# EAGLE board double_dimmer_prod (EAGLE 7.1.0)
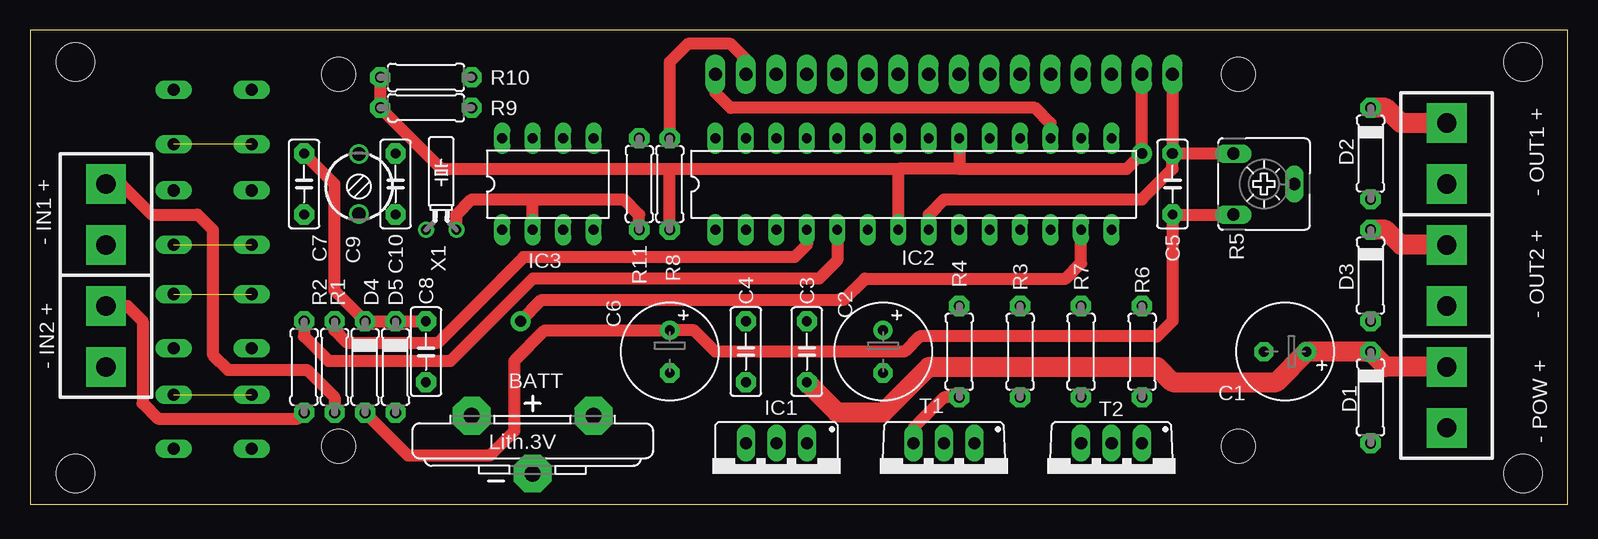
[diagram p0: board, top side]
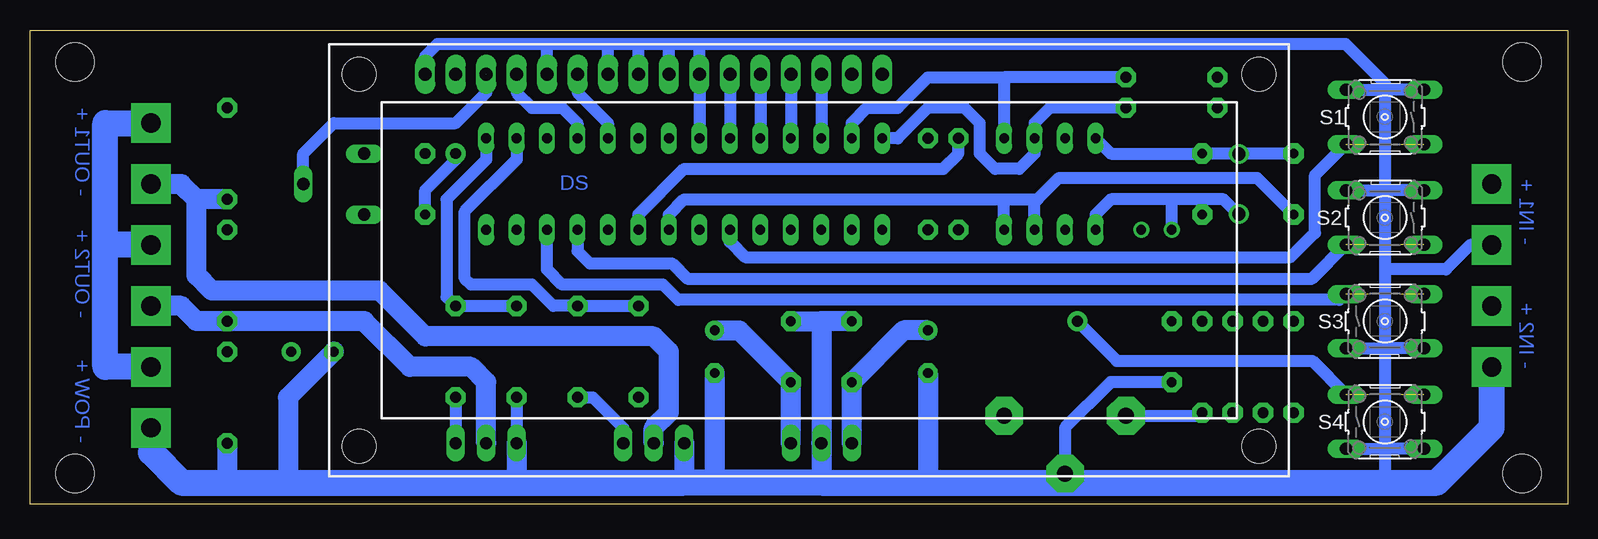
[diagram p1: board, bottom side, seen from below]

Size 128.18 x 39.51 mm. Coordinates in mm from the lower left corner, seen from the top.
Outline: 128.18,0 128.18,39.51 0,39.51 0,0 128.18,0
Copper layers (1*16): Top 0.035mm / dielectric 1.5mm / Bottom 0.035mm
Design rules "default": minimum track width 10mil, minimum drill 24mil, track to track 8mil, track to pad 8mil, pad to pad 8mil, via to via 8mil, smd to smd 8mil, copper to edge 40mil, drill to drill 8mil, minimum pad ring 10mil, minimum via ring 8mil, stop-mask expansion 4mil, vias tented up to drill 0mil, thermal gap 10mil
Holes 3.2 mm at 3.8,36.83 3.8,2.54 124.45,2.54 124.45,36.83

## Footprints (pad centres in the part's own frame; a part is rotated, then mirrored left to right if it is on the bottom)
CR2032V = drill 1.321 pad 3.15 octagon: + -2.54,-5.08; +@1 -2.54,5.08; - 2.286,0
E3,5-8 = drill 0.813 pad 1.6: + -1.778,0 | drill 0.813 pad 1.6 octagon: - 1.778,0
C050-025X075 = drill 0.813 pad 1.676 octagon: 1 -2.54,0; 2 2.54,0
CTRIM3050.504 = drill 1.1: 1 -2.5,0; 2 2.5,0
0207/7 = drill 0.9 pad 1.676 octagon: 1 -3.81,0; 2 3.81,0
78XXS = drill 1.016 long: GND 0,-2.54; IN -2.54,-2.54; OUT 2.54,-2.54
DIL28-3 = drill 0.813 long: 1 -16.51,-3.81; 2 -13.97,-3.81; 3 -11.43,-3.81; 4 -8.89,-3.81; 5 -6.35,-3.81; 6 -3.81,-3.81; 7 -1.27,-3.81; 8 1.27,-3.81; 9 3.81,-3.81; 10 6.35,-3.81; 11 8.89,-3.81; 12 11.43,-3.81; 13 13.97,-3.81; 14 16.51,-3.81; 15 16.51,3.81; 16 13.97,3.81; 17 11.43,3.81; 18 8.89,3.81; 19 6.35,3.81; 20 3.81,3.81; 21 1.27,3.81; 22 -1.27,3.81; 23 -3.81,3.81; 24 -6.35,3.81; 25 -8.89,3.81; 26 -11.43,3.81; 27 -13.97,3.81; 28 -16.51,3.81
DIL08 = drill 0.813 long: 1 -3.81,-3.81; 2 -1.27,-3.81; 3 1.27,-3.81; 4 3.81,-3.81; 5 3.81,3.81; 6 1.27,3.81; 7 -1.27,3.81; 8 -3.81,3.81
LCD-16X2 = drill 1.1 long: 1 -32,15.5; 2 -29.46,15.5; 3 -26.92,15.5; 4 -24.38,15.5; 5 -21.84,15.5; 6 -19.3,15.5; 7 -16.76,15.5; 8 -14.22,15.5; 9 -11.68,15.5; 10 -9.14,15.5; 11 -6.6,15.5; 12 -4.06,15.5; 13 -1.52,15.5; 14 1.02,15.5; 15 3.56,15.5; 16 6.1,15.5 | hole 2.8: -37.5,15.5; -37.5,-15.5; 37.5,15.5; 37.5,-15.5
CA6V = drill 1.016 long: A -2.54,-2.54; E 2.54,-2.54; S 0,2.54
B3F-10XX = drill 1.016 long: 1 -3.251,2.261; 2 3.251,2.261; 3 -3.251,-2.261; 4 3.251,-2.261
TO220BV = drill 1.016 long: D 0,-2.54; G -2.54,-2.54; S 2.54,-2.54
TC26H = drill 0.813: 1 -1.27,0; 2 1.27,0

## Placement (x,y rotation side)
BATT  [CR2032V]  41.9,4.83 270 top
C1  220uF  [E3,5-8]  104.64,12.7 180 top
C2  220uF  [E3,5-8]  71.11,12.7 270 top
C3  100nF  [C050-025X075]  64.76,12.7 90 top
C4  100nF  [C050-025X075]  59.68,12.7 90 top
C5  100nF  [C050-025X075]  95.24,26.67 90 top
C6  220uF  [E3,5-8]  53.33,12.7 270 top
C7  100nF  [C050-025X075]  22.85,26.67 270 top
C8  100nF  [C050-025X075]  33.01,12.7 270 top
C9  22pF  [CTRIM3050.504]  27.42,26.67 270 top
C10  22pF  [C050-025X075]  30.47,26.67 270 top
D1  1N5819  [0207/7]  111.75,8.89 90 top
D2  1N5819  [0207/7]  111.75,29.21 90 top
D3  1N5819  [0207/7]  111.75,19.05 90 top
D4  1N5819  [0207/7]  27.93,11.43 270 top
D5  1N5819  [0207/7]  30.47,11.43 270 top
IC1  7805  [78XXS]  62.22,2.54 180 top
IC2  ATMEGA8  [DIL28-3]  73.65,26.67 0 top
IC3  PFC8583  [DIL08]  43.17,26.67 0 top
IC4  LCD2x16  [LCD-16X2]  63.24,20.32 0 bottom
R1  3.3k  [0207/7]  25.39,11.43 270 top
R2  3.3k  [0207/7]  22.85,11.43 270 top
R3  47R  [0207/7]  82.54,12.7 90 top
R4  3.3k  [0207/7]  77.46,12.7 90 top
R5  10k  [CA6V]  102.86,26.67 270 top
R6  47R  [0207/7]  92.7,12.7 90 top
R7  3.3k  [0207/7]  87.62,12.7 90 top
R8  47R  [0207/7]  53.33,26.67 270 top
R9  3.3k  [0207/7]  33.01,33.02 0 top
R10  3.3k  [0207/7]  33.01,35.56 0 top
R11  1M  [0207/7]  50.79,26.67 270 top
S1  [B3F-10XX]  15.23,32.26 180 bottom
S2  [B3F-10XX]  15.23,23.88 180 bottom
S3  [B3F-10XX]  15.23,15.24 0 bottom
S4  [B3F-10XX]  15.23,6.86 0 bottom
T1  [TO220BV]  76.19,2.54 180 top
T2  [TO220BV]  90.16,2.54 180 top
X1  32kHz  [TC26H]  34.28,22.86 0 top

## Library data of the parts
BATT = battery
C1-C10 D1-D5 R1-R4 R6-R11 = rcl
IC1 = v-reg
IC2 = avr-4
IC3 = micro-philips; OC_FARNELL: unknown; OC_NEWARK: unknown
IC4 = moja2
R5 = pot
S1-S4 = switch-omron; MPN: B3F-1000; OC_FARNELL: 176432; OC_NEWARK: 36M3542
T1 T2 = transistor-power
X1 = crystal; OC_FARNELL: unknown; OC_NEWARK: unknown

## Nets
32K: IC2.9 R11.1
BKL: IC2.17 IC4.16
D4: IC2.23 IC4.11
D5: IC2.24 IC4.12
D6: IC2.25 IC4.13
D7: IC2.26 IC4.14
EIN1: IC2.4 R1.1
EIN2: IC2.5 R2.1
EN: IC2.19 IC4.6
GND: BATT.- C1.- C2.- C3.2 C4.2 C5.2 C6.- C7.2 C8.2 D1.1 IC1.GND IC2.8 IC2.22 IC3.3 IC3.4 IC4.1 IC4.5 IC4.7 IC4.8 IC4.9 IC4.10 R4.1 R5.A R7.1 S1.3 S1.4 S2.3 S2.4 S3.3 S3.4 S4.3 S4.4 T1.S T2.S
N$1: R6.1 T2.G
N$2: D2.1 T1.D
N$3: IC4.3 R5.S
N$4: D3.1 T2.D
N$5: R3.1 T1.G
N$6: BATT.+ D5.2
N$7: IC4.15 R8.1
N$8: C9.2 C10.2 IC3.1 X1.1
N$9: R2.2
N$10: IC3.2 R11.2 X1.2
N$11: R1.2
N$40: C7.1 C8.1 C9.1 C10.1 D4.1 D5.1 IC3.8
OT1: IC2.16 R3.2 R4.2
OT2: IC2.15 R6.2 R7.2
RS: IC2.18 IC4.4
RXD: IC2.2
SCL: IC2.28 IC3.6 R9.2
SDA: IC2.27 IC3.5 R10.2
SW1: IC2.6 S1.1 S1.2
SW2: IC2.11 S2.1 S2.2
SW3: IC2.12 S3.1 S3.2
SW4: IC2.13 S4.1 S4.2
TXD: IC2.3
VCC: C1.+ C2.+ C3.1 D1.2 D2.2 D3.2 IC1.IN
VDD: C4.1 C5.1 C6.+ D4.2 IC1.OUT IC2.7 IC2.20 IC4.2 R5.E R8.2 R9.1 R10.1

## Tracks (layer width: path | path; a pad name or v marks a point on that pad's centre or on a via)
32K
  Bottom 1.016: IC2.9 77.46,24.13 73.65,27.94 52.06,27.94 50.79,29.21 R11.1
BKL
  Top 1.016: IC2.17 85.08,31.75 83.81,33.02 58.41,33.02 57.14,34.29 IC4.16
D4
  Bottom 1.016: IC4.11 IC2.23
D5
  Bottom 1.016: IC4.12 IC2.24
D6
  Bottom 1.016: IC4.13 IC2.25
D7
  Bottom 1.016: IC4.14 IC2.26
EIN1
  Top 1.016: R1.1 25.39,14.48 26.41,13.46 34.03,13.46 41.14,20.57 63.74,20.57 64.76,21.59 IC2.4
EIN2
  Top 1.016: R2.1 22.85,13.97 24.88,11.94 35.04,11.94 41.9,18.8 65.78,18.8 67.3,20.32 IC2.5
EN
  Bottom 1.016: IC4.6 82.54,34.29 80,31.75 IC2.19
GND  (via drill 0.9 pad 1.68, 1.6 pad 3.3)
  Top 1.016: R5.A C5.2 | IC4.1 C5.2 95.24,27.94 92.69,25.4 76.19,25.4 74.92,24.13 IC2.8 | R4.1 76.19,8.89 73.65,6.35 T1.S
  Bottom 1.016: 15.23,34.8 15.23,35.05 18.53,38.35 72.38,38.35 | 15.23,34.8 15.23,26.16 | 15.23,26.16 15.23,25.91 | 15.23,25.91 15.23,19.56 | 15.23,19.56 15.23,13.21 | 15.23,13.21 15.23,12.95 | 15.23,12.95 15.23,4.57 | 15.23,4.57 15.23,4.32 | 15.23,4.32 15.23,2.03 14.98,1.78 | S3.3 15.46,12.98 15.23,13.21 | S3.4 15.21,12.98 15.23,12.95 | S4.4 15.21,4.6 15.23,4.57 | S4.3 15.51,4.6 15.23,4.32 | 72.38,38.35 IC4.10 IC2.22 | IC4.7 80,38.1 | 80,38.1 80,38.35 77.46,38.35 | 77.46,38.35 74.92,38.35 | 74.92,38.35 72.38,38.35 | IC4.9 74.92,38.35 | IC4.8 77.46,38.35 | IC4.1 95.24,37.33 94.22,38.35 85.08,38.35 | 85.08,38.35 80.25,38.35 80,38.1 | IC4.5 85.08,38.35 | C5.2 | R7.1 T2.S | C7.2 25.9,27.18 42.41,27.18 44.19,25.4 44.44,25.4 | S1.3 14.95,34.52 15.23,34.8 | S1.4 15.51,34.52 15.23,34.8 | S2.3 15,26.14 15.23,25.91 | S2.4 15.25,26.14 15.23,26.16 | C8.2 38.09,10.16 41.9,6.35 BATT.- | v6.34,21.59 8.12,21.59 10.15,19.56 15.23,19.56 | IC2.8 74.92,24.13 73.65,25.4 46.98,25.4 | 46.98,25.4 44.44,25.4 | IC3.3 44.44,25.4 | IC3.4 46.98,25.4
  Bottom 1.676: 62.22,1.78 IC1.GND 62.22,15.24 | T1.S 73.65,1.78 | T2.S 87.62,1.78 | D1.1 111.75,1.78 | C1.- 106.67,8.89 106.67,2.03 106.92,1.78 | C2.- 71.11,1.78 | C3.2 62.22,15.24 | C4.2 62.22,15.24 | C6.- 53.33,1.78
  Bottom 2.184: v118.1,6.35 118.1,4.32 115.56,1.78 111.75,1.78 106.92,1.78 87.62,1.78 73.65,1.78 71.11,1.78 62.22,1.78 53.33,1.78 41.9,1.78 | 41.9,1.78 14.98,1.78 10.91,1.78 6.34,6.35 v6.34,11.43 | BATT.- 41.9,1.78
  other vias: 95.24,29.21
N$1
  Bottom 1.016: R6.1 T2.G
N$2  (via drill 1.6 pad 3.3)
  Bottom 1.676: T1.D 76.19,6.35 74.92,7.62 74.92,12.7 76.19,13.97 95.24,13.97 99.05,17.78 113.02,17.78 114.29,19.05 114.29,25.4 | 114.29,25.4 115.56,26.67 v118.1,26.67 | D2.1 114.29,25.4
N$3  (1 unrouted)
  Bottom 1.016: R5.S 105.4,29.21 102.86,31.75 92.7,31.75 90.16,34.29 IC4.3
N$4  (via drill 1.6 pad 3.3)
  Bottom 1.676: T2.D 90.16,10.16 91.43,11.43 96.51,11.43 100.32,15.24 D3.1 114.29,15.24 115.56,16.51 v118.1,16.51
N$5
  Bottom 1.016: R3.1 81.27,8.89 78.73,6.35 T1.G
N$6
  Bottom 1.016: BATT.+ 30.72,7.37 D5.2
N$7
  Top 1.016: IC4.15 59.68,37.09 58.41,38.35 54.85,38.35 53.33,36.83 R8.1
N$8
  Bottom 1.016: C9.2 27.42,24.13 28.69,25.4 30.47,25.4 | 30.47,25.4 33.01,25.4 | 33.01,25.4 38.09,25.4 39.36,24.13 IC3.1 | C10.2 30.47,25.4 | X1.1 33.01,25.4
N$9  (via drill 1.6 pad 3.3)
  Top 1.016: v6.34,16.51 8.12,16.51 9.39,15.24 9.39,8.38 10.66,7.11 22.34,7.11 R2.2
N$10
  Top 1.016: X1.2 35.55,24.13 36.82,25.4 41.9,25.4 | 41.9,25.4 49.52,25.4 50.79,24.13 R11.2 | IC3.2 41.9,25.4
N$11  (via drill 1.6 pad 3.3)
  Top 1.016: R1.2 25.39,8.89 23.1,11.18 16.5,11.18 15.23,12.45 15.23,22.86 13.96,24.13 10.15,24.13 7.61,26.67 v6.34,26.67
N$40
  Top 1.016: C8.1 D5.1 D4.1 25.39,17.78 25.39,26.67 C7.1
  Bottom 1.016: IC3.8 38.09,29.21 C10.1 27.42,29.21 | C7.1 27.42,29.21 | C9.1 27.42,29.21
OT1
  Bottom 1.016: R4.2 R3.2 84.57,16.51 86.35,18.29 91.43,18.29 91.94,18.8 91.94,24.38 87.62,28.7 IC2.16
OT2
  Bottom 1.016: R7.2 R6.2 93.46,17.27 93.46,25.4 90.16,28.7 IC2.15
RS
  Bottom 1.016: IC4.4 87.62,34.29 86.35,33.02 83.81,33.02 82.54,31.75 IC2.18
SCL
  Bottom 1.016: R9.2 43.17,33.02 44.44,31.75 IC3.6 44.44,29.21 45.71,27.94 47.74,27.94 49.01,29.21 49.01,31.75 50.28,33.02 53.33,33.02 55.87,30.48 IC2.28
SDA
  Bottom 1.016: IC2.27 59.68,31.75 58.41,33.02 55.87,33.02 53.33,35.56 46.98,35.56 | 46.98,35.56 IC3.5 | R10.2 46.98,35.56
SW1  (1 unrouted)
  Bottom 1.016: IC2.6 69.84,21.84 68.57,20.57 23.1,20.57 21.07,22.61 21.07,27.41 S1.2
SW2  (1 unrouted)
  Bottom 1.016: IC2.11 82.54,21.08 81.52,20.07 74.67,20.07 73.4,18.8 21.3,18.8 S2.2
SW3  (1 unrouted)
  Bottom 1.016: S3.1 18.51,17.5 19.04,17.02 74.16,17.02 75.43,18.29 83.81,18.29 85.08,19.56 IC2.12
SW4  (via drill 0.9 pad 1.68)  (1 unrouted)
  Top 1.016: v40.88,15.24 42.66,17.02 67.81,17.02 69.59,18.8 86.35,18.8 87.62,20.07 IC2.13
  Bottom 1.016: v40.88,15.24 37.58,11.94 21.3,11.94 S4.1
VCC  (via drill 1.6 pad 3.3)
  Top 1.676: v118.1,31.75 114.29,31.75 113.02,33.02 D2.2 | v118.1,21.59 114.29,21.59 113.02,22.86 D3.2 | v118.1,11.43 113.02,11.43 D1.2 C1.+ 103.88,10.16 95.24,10.16 93.97,11.43 74.92,11.43 71.11,7.62 67.3,7.62 C3.1
  Bottom 1.676: IC1.IN C3.1 69.08,14.48 C2.+
  Bottom 2.184: v118.1,11.43 121.91,11.43 121.91,21.84 | 121.91,21.84 121.91,31.75 v118.1,31.75 | v118.1,21.59 121.66,21.59 121.91,21.84
VDD  (via drill 0.9 pad 1.68)
  Top 1.016: R10.1 R9.1 34.28,27.94 53.33,27.94 | 53.33,27.94 72.38,27.94 | IC2.20 77.46,27.94 | 77.46,27.94 72.38,27.94 | IC2.7 72.38,27.94 | D4.2 31.49,4.06 38.34,4.06 40.38,6.1 40.38,11.94 42.92,14.48 C6.+ 55.36,14.48 57.14,12.7 72.89,12.7 74.16,13.97 93.97,13.97 95.24,15.24 C5.1 R5.E | 77.46,27.94 91.43,27.94 v92.7,29.21 IC4.2 | R8.2 53.33,27.94
  Bottom 1.016: C5.1 95.24,26.16 92.7,28.7 v92.7,29.21
  Bottom 1.676: IC1.OUT C4.1 55.36,14.48 C6.+

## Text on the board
Bottom: DS | - OUT1 + | - IN1 + | - IN2 + | - OUT2 + | - POW +
tPlace: - OUT1 + | - IN1 + | - IN2 + | - OUT2 + | - POW +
